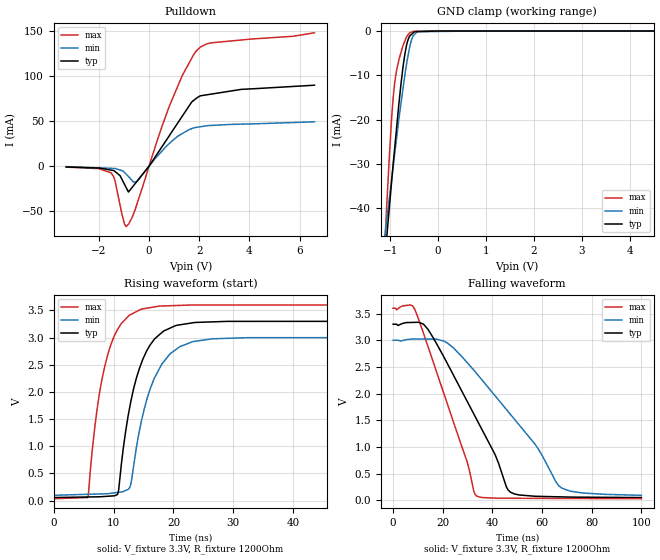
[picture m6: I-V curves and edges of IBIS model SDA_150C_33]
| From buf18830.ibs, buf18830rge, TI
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[Model] SDA_150C_33
|Signals SDA(15)
Model_type   I/O_open_drain
Polarity   Non-Inverting
Enable   Active-Low
Vinl = 0.99
Vinh = 2.31
Vmeas = 1.65
Vref = 1.65
Cref = 0pF
Rref = 10000
| Rpullup to DVDD = 1k
|   typ   min   max
|   (nom PVT)   (slow PVT)   (Fast PVT)
|   Output Low
|C_comp   1.0141E-12   8.35757E-13   1.26497E-12
|   Output High
C_comp   1.13784E-12   9.81932E-13   1.30641E-12
| Where   nom PVT is  Nominal Process, 3.3V, 57C
|   Fast PVT is Strong Process, 3.6V, -40C
|   Slow PVT is Weak Process, 3.0V, 125C
[Model Spec]   |3.3V model
Vinl   0.99   0.9   1.08
Vinh   2.31   2.1   2.52
|Vinl = 0.3 X DVDD
|Vinh = 0.7 X DVDD
[Voltage Range]   3.3   3   3.6
|Operating Temperature   27   85   -40
[Temperature Range]   92   150   -40
[Pullup Reference]   3.3   3   3.6
[Pulldown Reference]   0   0   0
[Power Clamp Reference]   3.3   3   3.6
[GND Clamp Reference]   0   0   0
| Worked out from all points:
|   slope of the pulldown table from 0 to 0.495 V, typ, clamps not added: 23.9 ohm
|   GND clamp passes 1 mA (typ) near -0.58 V on its own axis
|   falling waveform, V_fixture 3.3V, R_fixture 1200Ohm: 20-80 % time 21.6ns typ, 29ns min, 15.6ns max; typ from 3.3 V to 0.055 V
|   rising waveform, V_fixture 3.3V, R_fixture 1200Ohm: 20-80 % time 3.76ns typ, 4.21ns min, 3.33ns max; typ from 0.055 V to 3.3 V
[Pulldown]
|   Voltage   I(typ)   I(min)   I(max)
-3.3V     -923.4uA   -611.3uA   -1.057mA
-1.508V   -4.431mA   -2.464mA   -7.667mA
-1.355V   -5.95mA    -2.622mA   -16.42mA
-1.095V   -13.83mA   -4.87mA    -51.39mA
-913.6mV  -23.71mA   -8.89mA    -66.93mA
-822mV    -28.69mA   -11.41mA   -64.33mA
-505.4mV  -17.66mA   -17.44mA   -43.99mA
828.8mV   34.63mA    25.57mA    67.83mA
1.329V    55.51mA    36.08mA    100.6mA
1.888V    75.2mA     42.92mA    127.6mA
2.489V    79.77mA    45.06mA    136.5mA
6.59V     89.56mA    49.05mA    147.6mA
[GND Clamp]
|   Voltage   I(typ)   I(min)   I(max)
-3.3V     -344.4mA   -259.6mA   -579.2mA
-1.121V   -52.58mA   -46.88mA   -49.92mA
-1.085V   -47.87mA   -43.62mA   -41.86mA
-1.066V   -45.47mA   -41.88mA   -37.62mA
-974.2mV  -34.24mA   -33.66mA   -20.14mA
-907.5mV  -26.31mA   -27.68mA   -11.61mA
-729mV    -7.696mA   -12.58mA   -3.153mA
-667.3mV  -3.544mA   -7.96mA    -1.486mA
-594.7mV  -1.106mA   -3.632mA   -394.2uA
-524mV    -451.3uA   -1.11mA    -103.1uA
-437.3mV  -138.9uA   -153uA     -34.96uA
6.59V     0A         0A         0A
[POWER Clamp]
|   SCR cell for ESD function. Effects occurr above VDD x 2
|   Voltage   I(typ)   I(min)   I(max)
-3.3V     0A         0A         0A
0V        0A         0A         0A
6.6V      0A         0A         0A
[Ramp]
R_load = 1200
|   typ   min   max
dV/dt_r   1.94704/3.75087e-009   1.74216/4.16553e-009   2.13988/3.33144e-009
dV/dt_f   1.94704/2.15554e-008   1.74216/2.90245e-008   2.13988/1.56234e-008
[Falling Waveform]
V_fixture = 3.3V
V_fixture_min = 3V
V_fixture_max = 3.6V
R_fixture = 1200Ohm
C_fixture = 0F
|   Time   V(typ)   V(min)   V(max)
0s        3.3V       3V         3.6V
8.776ns   3.334V     3.024V     3.574V
14.05ns   3.204V     3.022V     2.883V
20.56ns   2.678V     2.981V     1.986V
29.8ns    1.859V     2.584V     726.5mV
33.47ns   1.535V     2.389V     91.16mV
47.45ns   151mV      1.602V     41.49mV
58.46ns   77.36mV    966.5mV    39.82mV
67.85ns   67.65mV    235.5mV    38.4mV
100ns     54.93mV    96.39mV    33.53mV
[Rising Waveform]
V_fixture = 3.3V
V_fixture_min = 3V
V_fixture_max = 3.6V
R_fixture = 1200Ohm
C_fixture = 0F
|   Time   V(typ)   V(min)   V(max)
0s        54.93mV    96.39mV    33.53mV
5.697ns   65.15mV    114.5mV    56.04mV
7.646ns   68.64mV    120.7mV    1.984V
9.036ns   78.58mV    126.2mV    2.693V
10.64ns   112.7mV    149.3mV    3.146V
12.77ns   1.764V     261.2mV    3.418V
14.51ns   2.492V     1.396V     3.517V
18.03ns   3.089V     2.507V     3.58V
23.49ns   3.276V     2.93V      3.598V
100ns     3.3V       3V         3.6V
